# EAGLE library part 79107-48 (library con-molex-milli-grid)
RECEPTACAL
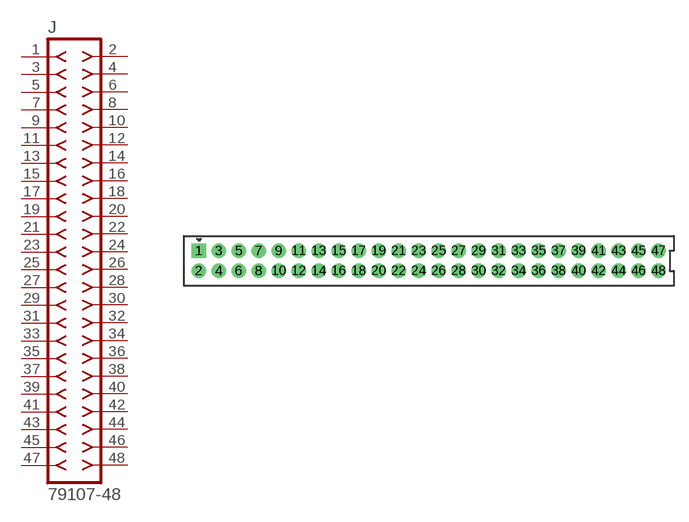
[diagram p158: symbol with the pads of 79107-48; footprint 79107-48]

Designator prefix J

## 79107-48  [79107-48]
1  1  pas
2  2  pas
3  3  pas
4  4  pas
5  5  pas
6  6  pas
7  7  pas
8  8  pas
9  9  pas
10  10  pas
11  11  pas
12  12  pas
13  13  pas
14  14  pas
15  15  pas
16  16  pas
17  17  pas
18  18  pas
19  19  pas
20  20  pas
21  21  pas
22  22  pas
23  23  pas
24  24  pas
25  25  pas
26  26  pas
27  27  pas
28  28  pas
29  29  pas
30  30  pas
31  31  pas
32  32  pas
33  33  pas
34  34  pas
35  35  pas
36  36  pas
37  37  pas
38  38  pas
39  39  pas
40  40  pas
41  41  pas
42  42  pas
43  43  pas
44  44  pas
45  45  pas
46  46  pas
47  47  pas
48  48  pas

## Footprint 79107-48 (pad centres in mm)
RECEPTACAL Dual Row, Vertical, Through-Hole
drill 0.914 square: 1 -23,1
drill 0.914: 2 -23,-1; 3 -21,1; 4 -21,-1; 5 -19,1; 6 -19,-1; 7 -17,1; 8 -17,-1; 9 -15,1; 10 -15,-1; 11 -13,1; 12 -13,-1; 13 -11,1; 14 -11,-1; 15 -9,1; 16 -9,-1; 17 -7,1; 18 -7,-1; 19 -5,1; 20 -5,-1; 21 -3,1; 22 -3,-1; 23 -1,1; 24 -1,-1; 25 1,1; 26 1,-1; 27 3,1; 28 3,-1; 29 5,1; 30 5,-1; 31 7,1; 32 7,-1; 33 9,1; 34 9,-1; 35 11,1; 36 11,-1; 37 13,1; 38 13,-1; 39 15,1; 40 15,-1; 41 17,1; 42 17,-1; 43 19,1; 44 19,-1; 45 21,1; 46 21,-1; 47 23,1; 48 23,-1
